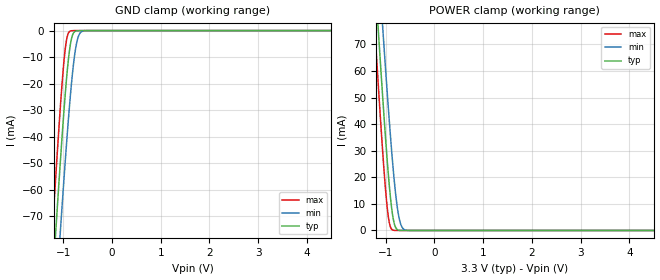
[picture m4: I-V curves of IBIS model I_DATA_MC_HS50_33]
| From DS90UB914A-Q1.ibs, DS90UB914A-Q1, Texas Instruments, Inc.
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|   Model I_DATA_MC_HS50_33
[Model]   I_DATA_MC_HS50_33
Model_type   Input
Vinl = 0.8V
Vinh = 2.0V
|   typ   min   max
|   (nom)   (weak)   (fast)
C_comp   0.5928pF   0.5928pF   0.5928pF
[Voltage Range]   3.300V   3.000V   3.600V
[Temperature Range]   25.0   105.0   -40.0
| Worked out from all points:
|   GND clamp passes 1 mA (typ) near -0.79 V on its own axis
|   POWER clamp passes 1 mA (typ) near -0.79 V on its own axis
[GND Clamp]
|   Voltage   I(typ)   I(min)   I(max)
-3.3V     -740.6mA   -745.8mA   -738.2mA
-1.231V   -98.09mA   -123.6mA   -77.79mA
-1.221V   -95.19mA   -120.8mA   -74.82mA
-1.171V   -80.8mA    -106.8mA   -60.15mA
-1.142V   -72.29mA   -98.42mA   -51.51mA
-1.063V   -50.2mA    -76.54mA   -29.57mA
-953.7mV  -22.68mA   -47.87mA   -6.122mA
-914.1mV  -14.41mA   -38.13mA   -1.959mA
-854.7mV  -5.303mA   -24.69mA   -170.5uA
-735.9mV  -135.9uA   -5.644mA   -12.73uA
-597.3mV  -4.686uA   -180uA     -6.308uA
6.59V     0A         0A         0A
[POWER Clamp]
|   Voltage   I(typ)   I(min)   I(max)
-3.3V     739mA      744.2mA    736.5mA
-1.231V   97.8mA     123.3mA    77.53mA
-1.221V   94.9mA     120.5mA    74.57mA
-1.171V   80.55mA    106.4mA    59.93mA
-1.142V   72.05mA    98.12mA    51.32mA
-1.063V   50.01mA    76.28mA    29.43mA
-953.7mV  22.55mA    47.67mA    6.052mA
-914.1mV  14.3mA     37.95mA    1.918mA
-854.7mV  5.242mA    24.55mA    149.9uA
-735.9mV  126.1uA    5.581mA    432.6nA
-597.3mV  604.6nA    174.2uA    0A
6.59V     0A         0A         0A
